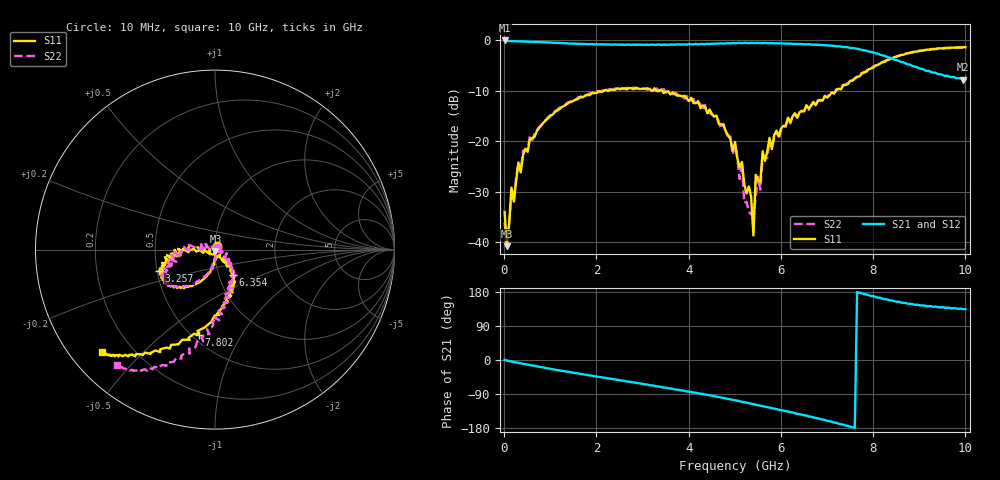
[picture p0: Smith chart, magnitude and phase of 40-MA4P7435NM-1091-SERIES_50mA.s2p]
!Agilent Technologies,E8364C,MY48140145,A.09.42.15
!Agilent E8364C: A.09.42.15
!Date: Wednesday, December 02, 2020 13:41:56
!Correction: S11(Full 2 Port(1,2))
!S21(Full 2 Port(1,2))
!S12(Full 2 Port(1,2))
!S22(Full 2 Port(1,2))
!S2P File: Measurements: S11, S21, S12, S22:
# Hz S  dB  R 50
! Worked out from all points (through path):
!   201 points, 10 MHz to 10 GHz, reference 50 ohm
!   highest |S21| = -0.09 dB at 10 MHz (marker M1); lowest = -7.8 dB at 9.95 GHz (marker M2)
!   group delay of S21, straight-line fit = 66.2 ps
!   lowest |S11| = -40.8 dB at 59.95 MHz (marker M3), VSWR 1.02, Z = 50.2 - j0.888 ohm
!   |S11| at or under -10 dB: start of sweep to 2.179 GHz; 3.299 GHz to 3.371 GHz (71.87 MHz wide, 2.16 % of centre); 3.424 GHz to 7.197 GHz (3.773 GHz wide, 71 % of centre)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
!   |S22| runs from -39.9 to -1.5 dB; largest |S21 - S12| = 0.028
!   S11 on the Smith chart (normalised r, x): 10 MHz: 1.02, +0.04; 3.257 GHz: 0.51, -0.14; 6.354 GHz: 1.17, -0.34; 7.802 GHz: 0.54, -0.67; 10 GHz: 0.09, -0.38
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1e7  -34.00 62.6  -0.09 0.7  -0.13 -0.9  -36.15 48.2
5.995e7  -40.77 -74.9  -0.18 -1.5  -0.17 -1.7  -39.90 -75.7
1.5985e8  -29.18 -81.6  -0.21 -4.2  -0.21 -4.3  -29.29 -81.4
2.098e8  -31.95 -79.8  -0.21 -5.4  -0.21 -5.4  -31.77 -87.0
3.097e8  -24.20 -90.6  -0.25 -7.7  -0.27 -7.8  -24.40 -88.8
5.5945e8  -19.49 -99.6  -0.34 -13.5  -0.34 -13.6  -18.99 -99.3
1.7083e9  -11.32 -129.9  -0.77 -38.0  -0.75 -37.7  -11.12 -132.9
3.25675e9  -9.55 -159.3  -0.94 -68.1  -0.90 -68.7  -10.07 -151.0
3.35665e9  -10.10 -160.7  -0.89 -70.0  -0.92 -70.6  -9.95 -151.4
4.35565e9  -13.23 -174.1  -0.85 -91.4  -0.81 -90.5  -12.84 -177.2
5.005e9  -20.15 172.4  -0.64 -106.4  -0.60 -106.4  -20.81 153.7
5.35465e9  -30.95 -85.6  -0.57 -115.0  -0.56 -115.0  -34.48 -41.4
5.4046e9  -38.65 -111.3  -0.58 -116.6  -0.56 -116.8  -34.63 53.0
5.45455e9  -26.68 -76.5  -0.60 -117.8  -0.59 -117.6  -31.04 -45.1
5.55445e9  -28.02 -59.2  -0.62 -120.7  -0.60 -120.6  -29.58 -13.3
5.6044e9  -22.00 -54.9  -0.62 -121.5  -0.63 -121.5  -23.03 -41.5
6.35365e9  -15.26 -53.8  -0.77 -141.9  -0.76 -141.8  -15.39 -59.1
6.7033e9  -12.23 -66.2  -0.92 -151.4  -0.90 -151.4  -12.49 -64.4
7.8022e9  -6.33 -100.8  -2.04 173.8  -1.97 174.5  -6.52 -96.6
8.35165e9  -3.78 -118.1  -3.49 157.4  -3.41 158.5  -3.84 -109.7
9.95005e9  -1.41 -137.2  -7.83 134.2  -7.73 135.2  -1.51 -129.9
1e10  -1.42 -137.6  -7.77 134.0  -7.76 133.9  -1.48 -130.3
